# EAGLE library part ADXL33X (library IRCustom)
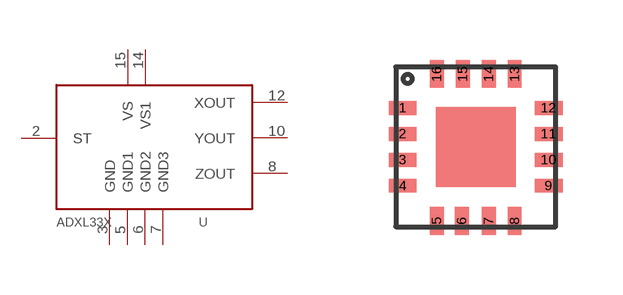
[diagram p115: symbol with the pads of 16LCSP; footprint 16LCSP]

Designator prefix -

## ADXL33X  [16LCSP]
2  ST  in
3  GND  sup
5  GND1  sup
6  GND2  sup
7  GND3  sup
8  ZOUT  out
10  YOUT  out
12  XOUT  out
14  VS1  sup
15  VS  sup

## Footprint 16LCSP (pad centres in mm)
smd 0.7 x 0.35: 1 -1.825,0.975; 2 -1.825,0.325; 3 -1.825,-0.325; 4 -1.825,-0.975; 9 1.825,-0.975; 10 1.825,-0.325; 11 1.825,0.325; 12 1.825,0.975
smd 0.35 x 0.7: 5 -0.975,-1.85; 6 -0.35,-1.85; 7 0.325,-1.85; 8 0.975,-1.85; 13 0.975,1.825; 14 0.325,1.825; 15 -0.325,1.825; 16 -0.975,1.825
